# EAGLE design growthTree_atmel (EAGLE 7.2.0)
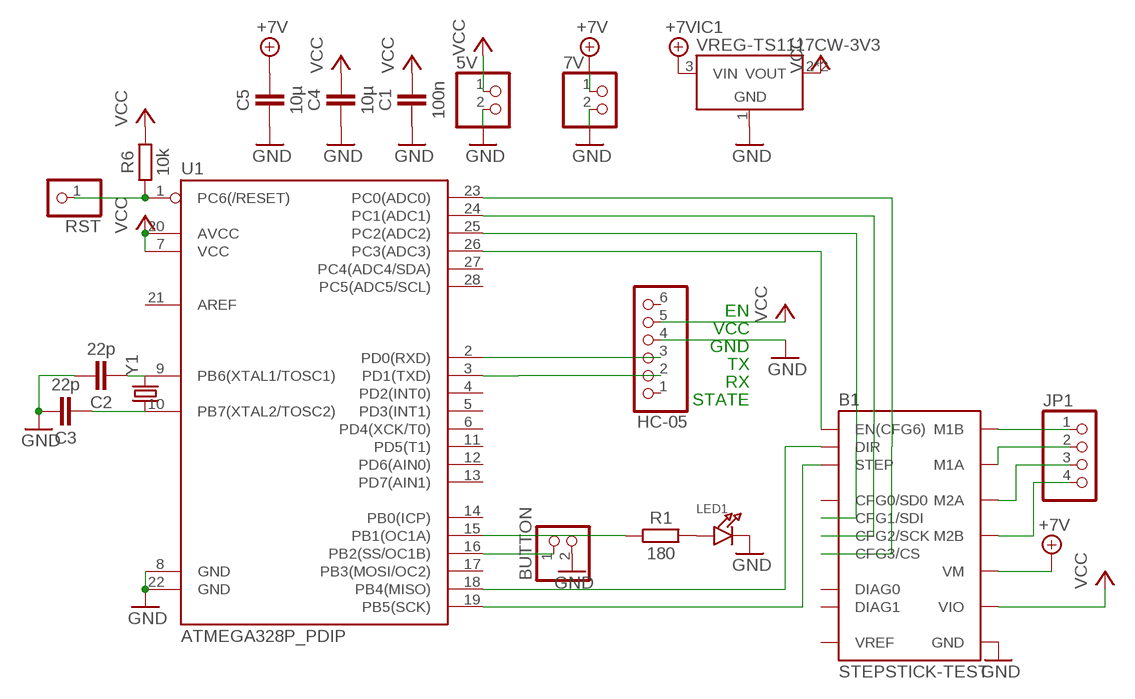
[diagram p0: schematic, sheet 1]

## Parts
5V  PINHD-1X2  [1X02]
7V  PINHD-1X2  [1X02]
B1  STEPSTICK-TEST  [STEPSTICK-TEST]
BUTTON  PINHD-1X2  [1X02]
C1  100n  CAPACITOR1206  [1206]
C2  22p  CAPACITOR  [603]
C3  22p  CAPACITOR  [603]
C4  10µ  CAPACITOR1206  [1206]
C5  10µ  CAPACITOR1206  [1206]
HC-05  PINHD-1X6  [1X06]
IC1  VREG-TS1117CW-3V3  [SOT223]
JP1  PINHD-1X4  [1X04]
LED1  LED1206  [CHIPLED_1206]
R1  180  RESISTOR1206  [1206]
R6  10k  RESISTOR1206  [1206]
RST  PINHD-1X1  [1X01]
U1  ATMEGA328P_PDIP  [DIL28-3]
Y1  CRYSTALHC49US  [HC49US]

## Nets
+7V: 7V.1 B1.VM C5.2 IC1.3(VIN)
GND: 5V.2 7V.2 B1.GND@1(GND) B1.GND@2(GND) BUTTON.2 C1.1 C2.2 C3.2 C4.1 C5.1 HC-05.4 IC1.1(GND) LED1.C U1.8(GND) U1.22(GND)
N$1: HC-05.3 U1.2(PD0(RXD))
N$2: HC-05.2 U1.3(PD1(TXD))
N$3: LED1.A R1.2
N$4: B1.M1B JP1.1
N$5: B1.M1A JP1.2
N$6: B1.M2A JP1.3
N$7: B1.M2B JP1.4
N$8: B1.CFG1(CFG1/SDI) U1.25(PC2(ADC2))
N$9: B1.CFG2(CFG2/SCK) U1.24(PC1(ADC1))
N$10: B1.CFG3(CFG3/CS) U1.23(PC0(ADC0))
N$11: R1.1 U1.15(PB1(OC1A))
N$12: BUTTON.1 U1.16(PB2(SS/OC1B))
N$13: B1.EN(EN(CFG6)) U1.26(PC3(ADC3))
N$14: R6.1 RST.1 U1.1(PC6(/RESET))
N$15: B1.STEP U1.19(PB5(SCK))
N$16: C2.1 U1.9(PB6(XTAL1/TOSC1)) Y1.2
N$17: C3.1 U1.10(PB7(XTAL2/TOSC2)) Y1.1
N$27: B1.DIR U1.18(PB4(MISO))
VCC: 5V.1 B1.VIO C1.2 C4.2 HC-05.5 IC1.2(VOUT) IC1.4(VOUT) R6.2 U1.7(VCC) U1.20(AVCC)
Unconnected: B1.DIAG0 B1.DIAG1 B1.NC/CFG0(CFG0/SD0) B1.VREF HC-05.1 HC-05.6 U1.4(PD2(INT0)) U1.5(PD3(INT1)) U1.6(PD4(XCK/T0)) U1.11(PD5(T1)) U1.12(PD6(AIN0)) U1.13(PD7(AIN1)) U1.14(PB0(ICP)) U1.17(PB3(MOSI/OC2)) U1.21(AREF) U1.27(PC4(ADC4/SDA)) U1.28(PC5(ADC5/SCL))

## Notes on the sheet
- EN
- VCC
- GND
- TX
- RX
- STATE

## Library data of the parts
5V 7V BUTTON = pinhead:PINHD-1X2: PIN HEADER
B1 = we-board:STEPSTICK: SilentStepStick - Trinamic TMC2100/TMC2130 Stepper Motor Driver TMC2100 - CFG pins for configuration TMC2130 - SPI for configuration Pin CFG0/SDO only available on TMC2130 SilentStepStick.
C1-C5 = thar:CAPACITOR
HC-05 = pinhead:PINHD-1X6: PIN HEADER
IC1 = we-power:VREG: Voltage Regulators (LDOs, Switching Converters...) LDOs Taiwan Semi TS1117 800mA max 15V - compatible On Semi NCP1117 1A max 20V - compatible Diodes AP2111H 0.6A max 6V (0.25V@0.6A) - compatible Diodes AP2114H 1A max 6V (0.45V@1A) Taiwan Semi TS9011 250mA max 12V - compatible Diodes AP2210 300mA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
JP1 = pinhead:PINHD-1X4: PIN HEADER
LED1 = microbuilder:LED: LED
R1 R6 = thar:RESISTOR
RST = pinhead:PINHD-1X1: PIN HEADER
U1 = SparkFun-DigitalIC:ATMEGA328P_PDIP: uC used in the Arduino 32kb flash, 1k EEPROM, 2k SRAM This is the through-hole version of this chip.
Y1 = SteveMarple:CRYSTAL: Crystals

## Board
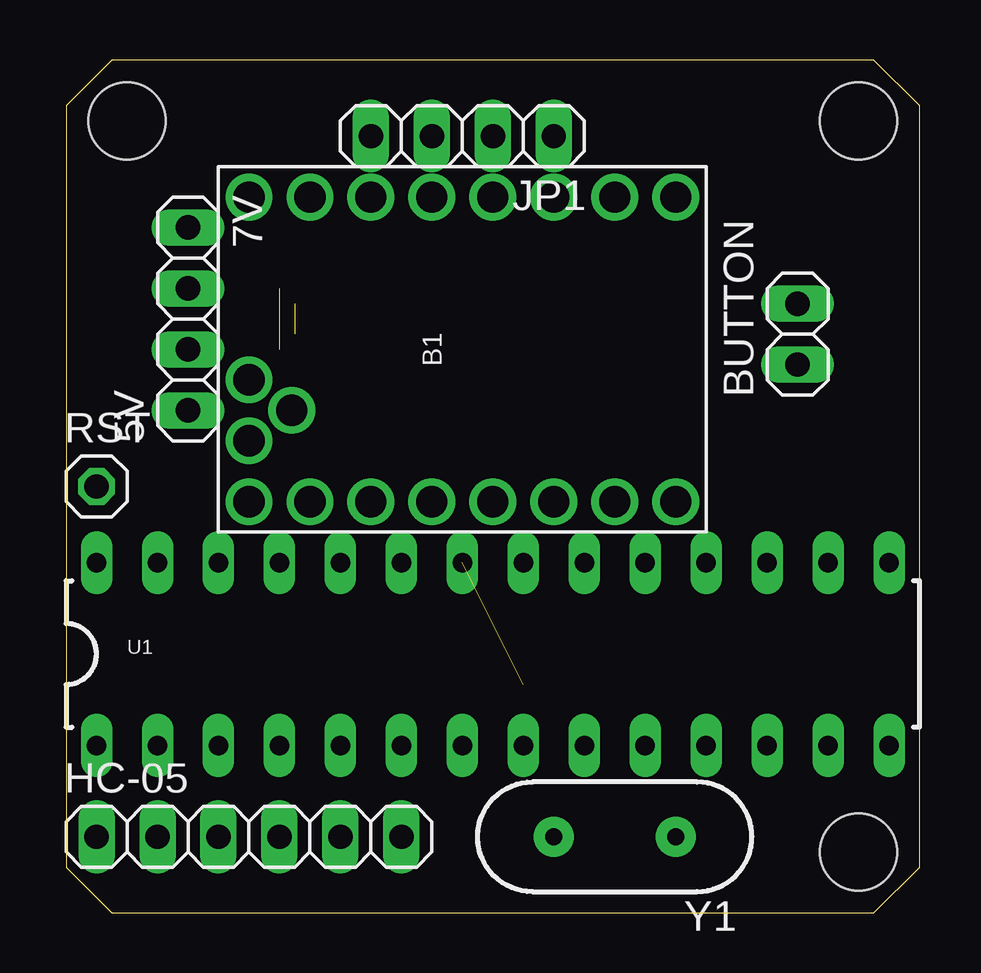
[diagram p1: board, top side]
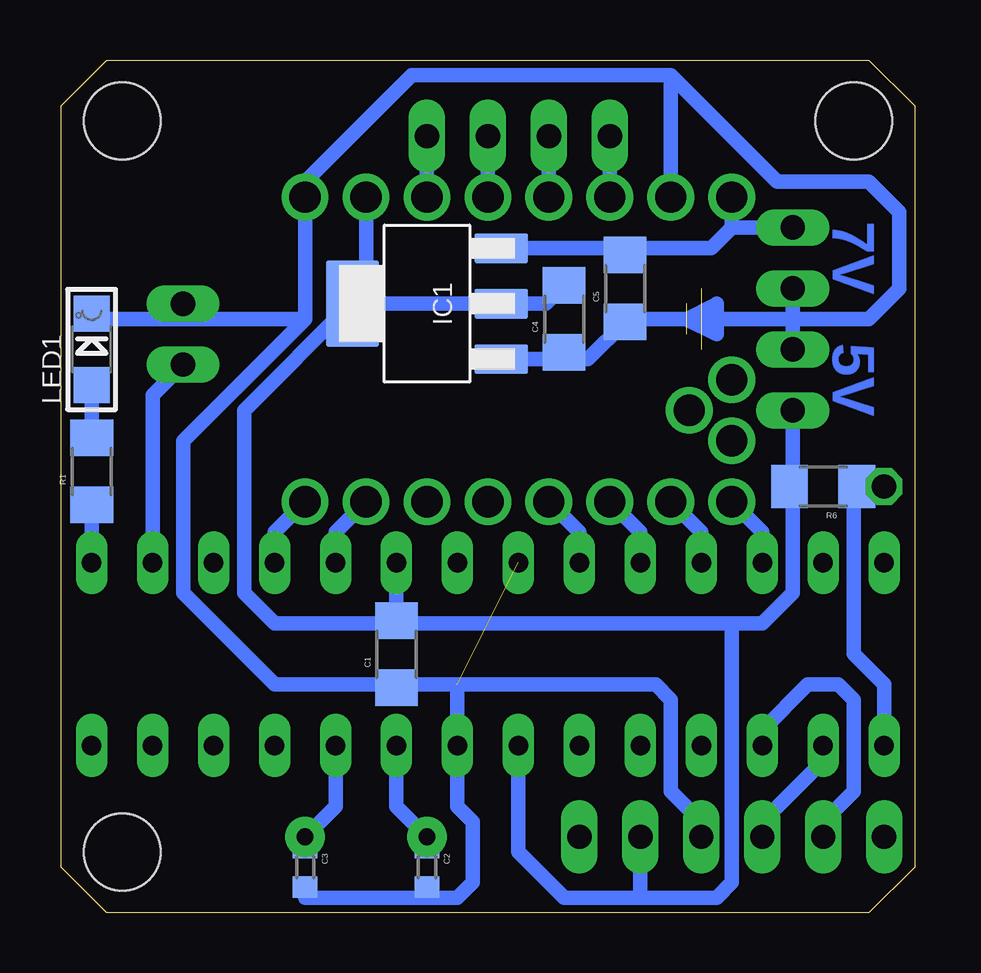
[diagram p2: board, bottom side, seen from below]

Size 35.56 x 35.56 mm. Coordinates in mm from the lower left corner, seen from the top.
Outline: 1.91,0 33.66,0 35.56,1.91 35.56,33.66 33.66,35.56 1.91,35.56 0,33.66 0,1.91 1.91,0
Copper layers (1*16): Top 0.035mm / dielectric 1.5mm / Bottom 0.035mm
Design rules "default": minimum track width 10mil, minimum drill 24mil, track to track 8mil, track to pad 8mil, pad to pad 8mil, via to via 8mil, smd to smd 8mil, copper to edge 40mil, drill to drill 8mil, minimum pad ring 10mil, minimum via ring 8mil, stop-mask expansion 4mil, vias tented up to drill 0mil, thermal gap 10mil
Holes 3.2 mm at 33.02,2.54 33.02,33.02 2.54,33.02

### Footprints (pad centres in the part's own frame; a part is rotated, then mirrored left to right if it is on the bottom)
1X02 = drill 1.016 long: 1 -1.27,0; 2 1.27,0
STEPSTICK-TEST = drill 1.3 pad 1.9: CFG1 -6.35,6.35; CFG2 -6.35,3.81; CFG3 -6.35,1.27; DIAG0 -2.54,7.112; DIAG1 -1.27,8.89; DIR -6.35,-8.89; EN -6.35,8.89; GND@1 6.35,6.35; GND@2 6.35,-8.89; M1A 6.35,-1.27; M1B 6.35,-3.81; M2A 6.35,1.27; M2B 6.35,3.81; NC -6.35,-3.81; NC/CFG0 -6.35,-1.27; STEP -6.35,-6.35; VIO 6.35,-6.35; VM 6.35,8.89; VREF -3.81,8.89
1206 = smd 1.524 x 1.778: 1 -1.397,0; 2 1.397,0
603 = smd 0.889 x 1.016: 1 -0.826,0; 2 0.826,0
1X06 = drill 1.016 long: 1 -6.35,0; 2 -3.81,0; 3 -1.27,0; 4 1.27,0; 5 3.81,0; 6 6.35,0
SOT223 = smd 2.235 x 1.219: 1 -3.099,2.311; 2 -3.099,0; 3 -3.099,-2.311 | smd 2.2 x 3.6: 4 3.099,0
1X04 = drill 1.016 long: 1 -3.81,0; 2 -1.27,0; 3 1.27,0; 4 3.81,0
CHIPLED_1206 = smd 1.5 x 1.5: A 0,-1.496; C 0,1.496
1X01 = drill 1.016 octagon: 1 0,0
DIL28-3 = drill 0.813 long: 1 -16.51,-3.81; 2 -13.97,-3.81; 3 -11.43,-3.81; 4 -8.89,-3.81; 5 -6.35,-3.81; 6 -3.81,-3.81; 7 -1.27,-3.81; 8 1.27,-3.81; 9 3.81,-3.81; 10 6.35,-3.81; 11 8.89,-3.81; 12 11.43,-3.81; 13 13.97,-3.81; 14 16.51,-3.81; 15 16.51,3.81; 16 13.97,3.81; 17 11.43,3.81; 18 8.89,3.81; 19 6.35,3.81; 20 3.81,3.81; 21 1.27,3.81; 22 -1.27,3.81; 23 -3.81,3.81; 24 -6.35,3.81; 25 -8.89,3.81; 26 -11.43,3.81; 27 -13.97,3.81; 28 -16.51,3.81
HC49US = drill 0.7 pad 1.651: 1 -2.54,0; 2 2.54,0

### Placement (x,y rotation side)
5V  5.08,22.23 90 top
7V  5.08,27.3 270 top
B1  16.51,23.49 90 top
BUTTON  30.48,24.13 90 top
C1  21.59,10.8 90 bottom
C2  20.32,1.91 270 bottom
C3  25.4,1.91 270 bottom
C4  14.61,24.77 90 bottom
C5  12.07,26.04 90 bottom
HC-05  7.62,3.18 0 top
IC1  20.32,25.4 180 bottom
JP1  16.51,32.38 180 top
LED1  34.29,23.49 0 bottom
R1  34.29,18.41 90 bottom
R6  3.81,17.78 180 bottom
RST  1.27,17.78 0 top
U1  17.78,10.8 0 top
Y1  22.86,3.18 180 top

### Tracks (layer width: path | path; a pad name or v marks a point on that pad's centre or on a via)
+7V
  Bottom 0.61: IC1.3 11.43,27.71 | 11.43,27.71 8.48,27.71 7.62,28.58 | 7V.1 6.35,28.58 7.62,28.58 | B1.VM 7.62,28.58 | C5.2 11.43,27.71
GND  (1 unrouted)
  Bottom 0.61: HC-05.4 8.89,3.81 10.16,5.08 10.16,8.89 10.79,9.52 19.05,9.52 | 20.32,0.64 19.05,0.64 18.42,1.27 18.42,3.81 19.05,4.45 U1.8 19.05,9.52 | 20.32,0.64 25.4,0.64 C3.2 | C2.2 20.32,0.64 | 10.16,32.38 B1.GND@1 10.16,32.38 | 10.16,32.38 10.16,33.02 | 10.16,33.02 10.16,32.38 | 19.05,9.52 21.46,9.52 C1.1 21.72,9.52 26.67,9.52 30.48,13.34 30.48,19.69 25.4,24.77 | 25.4,24.77 B1.GND@2 25.4,30.48 20.96,34.92 12.07,34.92 10.16,34.92 | LED1.C 34.06,24.99 34.06,24.77 34.29,24.77 30.48,24.77 | 5V.2 5.08,24.77 | 5.08,24.77 7V.2 | 30.48,24.77 25.4,24.77 | BUTTON.2 30.48,24.77 | 5.08,24.77 7.62,24.77 9.53,24.77 | 5.08,24.77 1.91,24.77 0.64,26.04 0.64,27.94 0.64,29.21 1.91,30.48 5.71,30.48 10.16,34.92 | 10.16,33.02 10.16,34.92 | 9.53,24.77 12.57,24.77 C5.1 13.61,23.09 14.61,23.09 | 14.96,23.09 C4.1 14.61,23.09 | IC1.1 14.61,23.09 | 9.53,24.77 8.25,25.4 8.25,24.13 9.53,24.77
N$1
  Bottom 0.61: U1.2 3.81,6.35 6.35,3.81 HC-05.3
N$2
  Bottom 0.61: U1.3 6.35,7.62 4.45,9.52 3.18,9.52 2.54,8.89 2.54,5.08 3.81,3.81 HC-05.2
N$3
  Bottom 0.61: R1.2 LED1.A
N$4
  Bottom 0.61: JP1.1 B1.M1B
N$5
  Bottom 0.61: JP1.2 B1.M1A
N$6
  Bottom 0.61: JP1.3 B1.M2A
N$7
  Bottom 0.61: JP1.4 B1.M2B
N$8
  Bottom 0.61: U1.25 8.89,15.88 B1.CFG1
N$9
  Bottom 0.61: U1.24 11.43,15.88 B1.CFG2
N$10
  Bottom 0.61: U1.23 13.97,15.88 B1.CFG3
N$11
  Bottom 0.61: U1.15 R1.1
N$12
  Bottom 0.61: U1.16 31.75,21.59 BUTTON.1
N$13
  Bottom 0.61: U1.26 6.35,15.88 B1.EN
N$14
  Bottom 0.61: U1.1 1.27,9.52 2.54,10.8 2.54,17.78 2.41,18.29 R6.1 RST.1
N$15
  Bottom 0.61: U1.19 24.13,15.88 B1.STEP
N$16
  Bottom 0.61: C2.1 Y1.2 21.59,4.45 U1.9
N$17
  Bottom 0.61: C3.1 Y1.1 24.13,4.45 U1.10
N$27
  Bottom 0.61: U1.18 26.67,15.88 B1.DIR
N$35  (1 unrouted)
N$36  (1 unrouted)
VCC
  Bottom 0.61: HC-05.5 11.43,1.91 11.43,0.64 | 11.43,0.64 14.61,0.64 16.51,2.54 U1.7 | U1.20 21.59,13.34 C1.2 | B1.VIO 22.86,26.04 23.5,25.4 | 23.5,25.4 27.94,20.95 27.94,13.34 26.67,12.06 21.46,12.06 | 21.46,12.06 21.08,12.06 C1.2 | R6.2 4.95,17.91 5.08,17.78 | 5.08,17.78 5.08,19.05 5.08,20.32 5V.1 | 5.08,17.78 5.08,13.34 6.35,12.06 7.62,12.06 | 7.62,12.06 21.46,12.06 | 21.46,12.06 C1.2 | 11.43,0.64 8.25,0.64 7.62,1.27 7.62,12.06 | 23.5,25.4 IC1.4 IC1.2 15.37,25.4 C4.2

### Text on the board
Bottom: 7V | 5V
